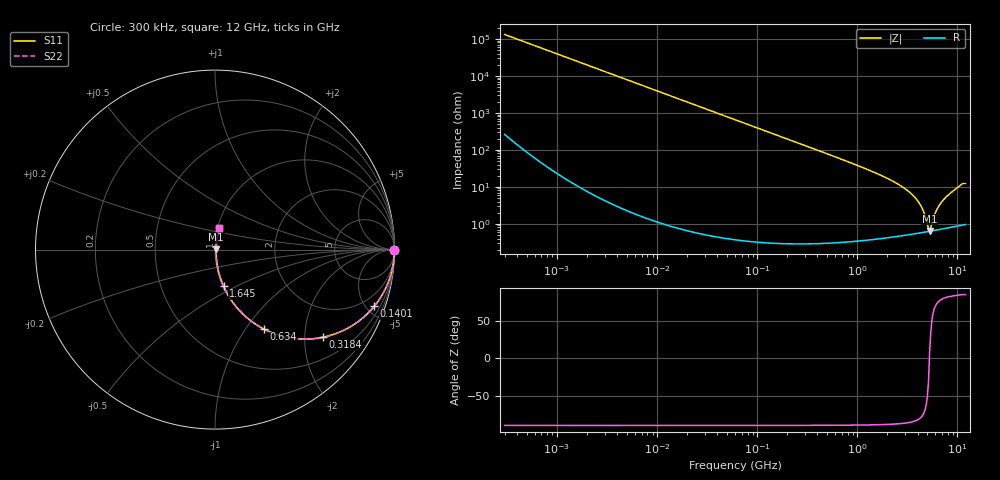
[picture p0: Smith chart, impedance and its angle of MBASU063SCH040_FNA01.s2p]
! MBASU063SCH040_FNA01  S-PARAMETER MODEL  ( Standard Model )
! Model Generated by TAIYO YUDEN Corporation (http://www.ty-top.com)
! Version 1.0
! TAIYO YUDEN Control No. 230609
! Copyright(c) 2023 TAIYO YUDEN CO.,LTD. All Rights Reserved.
! Product Description (link to TY-COMPAS)
! https://ds.yuden.co.jp/TYCOMPAS/or/detail?pn=MBASU063SCH040BFNA01&u=M
! Products Name : Multilayer Ceramic Capacitors
! Characteristics :
!  Capacitance : 4 [pF] , Rated Voltage : 50 [V] , TCC : CH / C0H
!  Case Size : 0.6 x 0.3 / 0.024 x 0.012 [mm/inch] , Thickness : 0.3 / 0.012 [mm/inch]
!  (Conditions: Temperature = 25 [degC] , DC Bias Voltage = 0 [V])
! External Node Assignments :
!  1  o---| |---o  2
! GND o---------o GND
! Frequency Range : 0.3MHz  -  12000MHz  [ 401 STEP ]
# MHZ S RI R 50
! Freq[MHz].  S11 Real  S11 Imag  S21 Real  S21 Imag  S12 Real  S12 Imag  S22 Real  S22 Imag
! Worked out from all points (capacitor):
!   401 points, 300 kHz to 12 GHz, reference 50 ohm
!   read as one part in series: C = 4.04 pF near 316.3 kHz
!   lowest |Z| = 639 mohm at 5.279 GHz (marker M1)
!   series resonance near 5.245 GHz, so ESL is about 230 pH
!   S11 on the Smith chart (normalised r, x): 300 kHz: open; 140.1 MHz: 1.01, -5.62; 318.4 MHz: 1.01, -2.46; 634 MHz: 1.01, -1.22; 1.645 GHz: 1.01, -0.43; 12 GHz: 1.02, +0.25
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0.3  1 -0.000762  2.1e-06 0.000762  2.1e-06 0.000762  1 -0.000762
1.769972  1 -0.0045  2.2e-05 0.0045  2.2e-05 0.0045  1 -0.0045
10.44266  0.9993 -0.0265  0.000711 0.0265  0.000711 0.0265  0.9993 -0.0265
60  0.9772 -0.149  0.0228 0.149  0.0228 0.149  0.9772 -0.149
140.0606  0.8872 -0.3158  0.1128 0.3158  0.1128 0.3158  0.8872 -0.3158
318.4019  0.6024 -0.4882  0.3976 0.4882  0.3976 0.4882  0.6024 -0.4882
353.9943  0.5504 -0.4962  0.4496 0.4962  0.4496 0.4962  0.5504 -0.4962
634.0297  0.2733 -0.4431  0.7267 0.4431  0.7267 0.4431  0.2733 -0.4431
994.7115  0.1293 -0.3311  0.8707 0.3311  0.8707 0.3311  0.1293 -0.3311
1645.489  0.0479 -0.2047  0.9521 0.2047  0.9521 0.2047  0.0479 -0.2047
2088.533  0.0285 -0.1536  0.9715 0.1536  0.9715 0.1536  0.0285 -0.1536
3026.31  0.0123 -0.0856  0.9877 0.0856  0.9877 0.0856  0.0123 -0.0856
3841.137  0.00766 -0.0473  0.9923 0.0473  0.9923 0.0473  0.00766 -0.0473
4385.161  0.00647 -0.0271  0.9935 0.0271  0.9935 0.0271  0.00647 -0.0271
4623.766  0.00624 -0.0192  0.9938 0.0192  0.9938 0.0192  0.00624 -0.0192
5006.236  0.00614 -0.00744  0.9939 0.00744  0.9939 0.00744  0.00614 -0.00744
5278.635  0.00624 0.00118  0.9938 -0.00118  0.9938 -0.00118  0.00624 0.00118
5565.855  0.00647 0.00823  0.9935 -0.00823  0.9935 -0.00823  0.00647 0.00823
6188.031  0.00723 0.0221  0.9928 -0.0221  0.9928 -0.0221  0.00723 0.0221
7064.448  0.0088 0.0399  0.9912 -0.0399  0.9912 -0.0399  0.0088 0.0399
10511.28  0.0195 0.1023  0.9805 -0.1023  0.9805 -0.1023  0.0195 0.1023
12000  0.0239 0.1185  0.9761 -0.1185  0.9761 -0.1185  0.0239 0.1185
